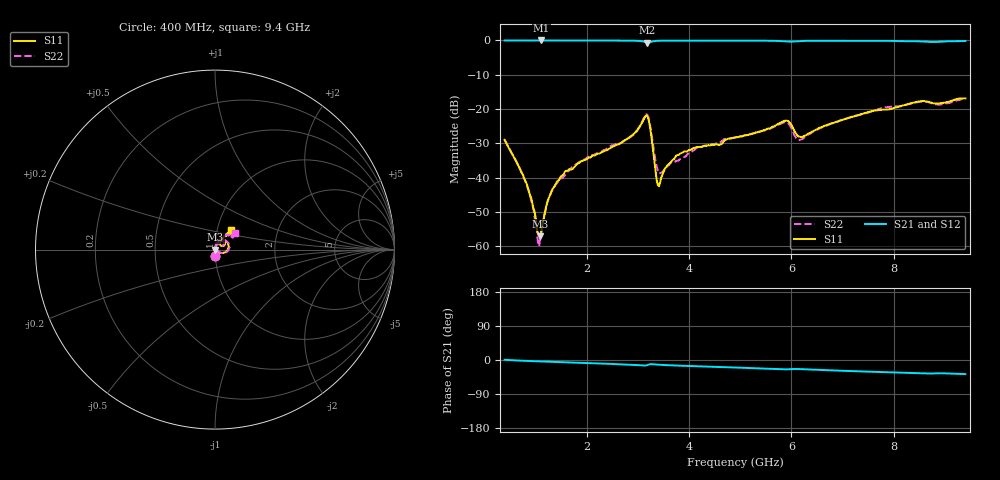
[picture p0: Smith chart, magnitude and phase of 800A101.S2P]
!  American Technical Ceramics  Date:  9/12/2007
!  One Norden Lane
!  Huntington Station,  NY.  11746-2102
!  Tel:  (631) 622-4700  Fax:  (631) 622-4748
!  Part Number  800A101  Mounting Orientation: Vertical
!  Description: Ultra Low ESR Microwave capacitors
!  Application: Coupling, Bypass, Tuning, DC Block
!  Filters, Matching
# GHZ S DB R 50
! Freq  |S11|  S11 Ph  |S21|  S21 Ph  |S12|  S12 Ph  |S22|  S22 Ph
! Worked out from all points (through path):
!   401 points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, 400 MHz to 9.4 GHz, reference 50 ohm
!   highest |S21| = -0.02 dB at 1.12 GHz (marker M1); lowest = -0.7 dB at 3.19 GHz (marker M2)
!   group delay of S21, straight-line fit = 11.4 ps
!   lowest |S11| = -57.2 dB at 1.098 GHz (marker M3), VSWR 1.00, Z = 50.1 + j0.0398 ohm
!   |S11| at or under -10 dB: start of sweep to end of sweep
!   |S22| runs from -60.0 to -16.9 dB; largest |S21 - S12| = 0.0066
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0.4  -29.00 -88.0  -0.02 0.6  -0.01 0.6  -28.98 -88.1
0.828  -41.71 -81.9  -0.02 -2.4  -0.01 -2.4  -42.09 -86.2
0.918  -45.88 -77.3  -0.02 -2.9  -0.01 -2.9  -46.80 -80.2
1.03  -55.22 -48.1  -0.02 -3.5  -0.01 -3.5  -55.21 -56.4
1.098  -57.17 16.6  -0.02 -3.8  -0.01 -3.9  -56.98 27.9
1.12  -55.33 37.5  -0.02 -3.9  -0.01 -4.0  -56.10 44.6
1.21  -48.54 64.9  -0.02 -4.4  -0.01 -4.4  -48.88 71.6
1.345  -43.11 72.6  -0.02 -5.0  -0.01 -5.1  -43.48 75.5
1.548  -39.14 75.9  -0.03 -6.0  -0.01 -6.1  -39.79 78.7
1.908  -35.14 75.7  -0.04 -7.6  -0.01 -7.7  -35.22 79.7
2.875  -27.87 71.0  -0.08 -12.4  -0.06 -12.5  -27.95 72.3
3.19  -22.10 11.9  -0.71 -13.2  -0.69 -13.3  -21.71 9.2
3.258  -27.06 -25.6  -0.45 -11.0  -0.42 -11.1  -26.27 -24.7
3.37  -40.73 -8.9  -0.14 -12.0  -0.12 -12.1  -36.69 -14.0
3.415  -42.54 31.4  -0.11 -12.5  -0.09 -12.6  -38.83 8.4
3.798  -33.44 76.8  -0.07 -14.8  -0.05 -15.0  -35.01 67.1
4.9  -28.31 68.3  -0.06 -19.9  -0.05 -20.0  -28.34 70.2
5.89  -23.42 41.0  -0.29 -24.6  -0.29 -24.9  -23.91 43.4
6.138  -28.01 32.6  -0.21 -23.9  -0.21 -24.1  -29.06 41.0
6.408  -26.61 54.1  -0.10 -25.4  -0.10 -25.7  -26.80 61.7
7.915  -20.10 51.6  -0.14 -32.6  -0.15 -32.9  -19.38 48.2
9.4  -16.89 50.5  -0.18 -37.2  -0.20 -37.5  -16.86 40.4
